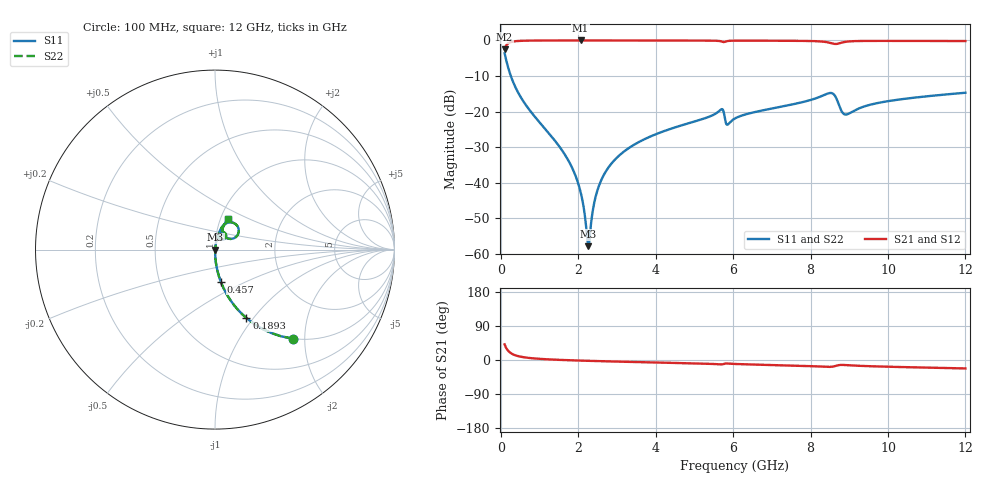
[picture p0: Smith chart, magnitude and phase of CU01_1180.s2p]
! S-parameter model data by Modelithics Inc. support@modelithics.com 813-866-6335 Tampa FL USA
! S-Parameter data specifications:
! Substrate: 20-mil Rogers, substrate thickness, H=0.508mm, Dielectric constant, Er=3.75
! PCB Mounting Pad Footprint: Pad width, PadW=0.35mm , Pad length, PadL=0.30mm , Pad gap, PadG (edge-to-edge)=0.25mm , Reference planes=0.85mm apart
! Created Wed May 09 13:18:57 2018
# hz S ma R 50
! 2 Port Network Data from SP1.SP block
! freq  magS11  angS11  magS21  angS21  magS12  angS12  magS22  angS22
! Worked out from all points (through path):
!   801 points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, 100 MHz to 12 GHz, reference 50 ohm
!   highest |S21| = -0.01 dB at 2.063 GHz (marker M1); lowest = -2.5 dB at 100 MHz (marker M2)
!   group delay of S21, straight-line fit = 6.78 ps
!   lowest |S11| = -57.9 dB at 2.257 GHz (marker M3), VSWR 1.00, Z = 50.1 - j0.0285 ohm
!   |S11| at or under -10 dB: 260.4 MHz to end of sweep
!   |S22| runs from -57.9 to -3.6 dB; largest |S21 - S12| = 0
!   S11 on the Smith chart (normalised r, x): 100 MHz: 1.00, -1.75; 189.2 MHz: 1.00, -0.92; 457 MHz: 1.00, -0.37; 12 GHz: 1.09, +0.38
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1e8  0.6597 -48.8  0.7511 41.2  0.7511 41.2  0.6597 -48.8
1.8925e8  0.419 -65.3  0.9075 24.6  0.9075 24.6  0.419 -65.3
4.57e8  0.1816 -79.8  0.9827 10.0  0.9827 10.0  0.1816 -79.8
1.661875e9  0.02449 -87.7  0.9986 -0.2  0.9986 -0.2  0.02449 -87.7
1.899875e9  0.01379 -86.2  0.9987 -1.1  0.9987 -1.1  0.01379 -86.2
2.0635e9  0.007341 -82.1  0.9987 -1.6  0.9987 -1.6  0.007341 -82.1
2.09325e9  0.00624 -80.5  0.9987 -1.7  0.9987 -1.7  0.00624 -80.5
2.256875e9  0.001278 -12.9  0.9987 -2.2  0.9987 -2.2  0.001278 -12.9
2.3015e9  0.001811 43.3  0.9987 -2.3  0.9987 -2.3  0.001811 43.3
2.39075e9  0.004463 70.6  0.9987 -2.6  0.9987 -2.6  0.004463 70.6
2.48e9  0.007271 76.8  0.9986 -2.8  0.9986 -2.8  0.007271 76.8
2.762625e9  0.01579 81.4  0.9985 -3.6  0.9985 -3.6  0.01579 81.4
3.268375e9  0.02963 82.2  0.998 -4.9  0.998 -4.9  0.02963 82.2
4.071625e9  0.04954 81.2  0.997 -6.8  0.997 -6.8  0.04954 81.2
5.678125e9  0.1059 67.8  0.9749 -11.5  0.9749 -11.5  0.1059 67.8
5.856625e9  0.0653 63.9  0.9791 -9.3  0.9791 -9.3  0.0653 63.9
6.05e9  0.07999 76.1  0.992 -10.5  0.992 -10.5  0.07999 76.1
8.04325e9  0.1476 69.9  0.9792 -16.3  0.9792 -16.3  0.1476 69.9
8.549e9  0.1817 47.5  0.9104 -17.8  0.9104 -17.8  0.1817 47.5
8.920875e9  0.09073 51.8  0.9585 -13.4  0.9585 -13.4  0.09073 51.8
1.002162e10  0.1404 70.2  0.985 -17.8  0.985 -17.8  0.1404 70.2
1.2e10  0.1837 66.7  0.9796 -22.2  0.9796 -22.2  0.1837 66.7
